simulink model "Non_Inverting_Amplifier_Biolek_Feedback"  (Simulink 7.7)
settings: Solver=ode113  StartTime=0.0  StopTime=10  RelTol=3e-14
libraries: fl_lib x7, nesl_utility x5, Memristor_lib x2

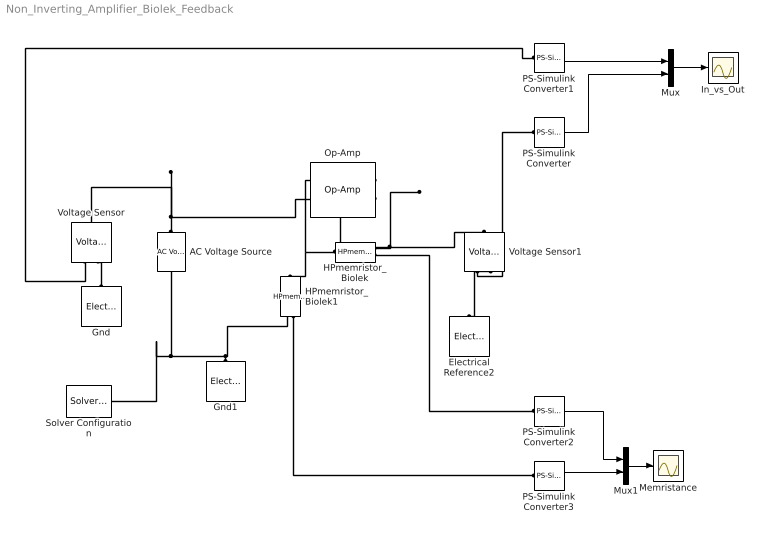
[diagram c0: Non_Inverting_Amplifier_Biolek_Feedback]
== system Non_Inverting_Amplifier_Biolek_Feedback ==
  AC Voltage Source : fl_lib/Electrical/Electrical Sources/AC Voltage Source  SystemSampleTime=-1  amp=1 V  shift=0 rad  omega=1 Hz  i_Log=off  v_Log=off  LocalVarNames=|i|v  LocalVarDescs=|i|v  LocalVarLogging=[0 0]
  Electrical Reference2 : fl_lib/Electrical/Electrical Elements/Electrical Reference  SystemSampleTime=-1  i_Log=off  LocalVarNames=|i  LocalVarDescs=|i  LocalVarLogging=0
  Gnd : fl_lib/Electrical/Electrical Elements/Electrical Reference  SystemSampleTime=-1  i_Log=off  LocalVarNames=|i  LocalVarDescs=|i  LocalVarLogging=0
  Gnd1 : fl_lib/Electrical/Electrical Elements/Electrical Reference  SystemSampleTime=-1  i_Log=off  LocalVarNames=|i  LocalVarDescs=|i  LocalVarLogging=0
  HPmemristor_Biolek : Memristor_lib/HPmemristor_Biolek  SystemSampleTime=-1  R_off=100 Ohm  R_on=2 Ohm  pp=10 m  u_v=1e-12 m^2/s/V  D=1e-8 m  w0=.01e-9 m  i_Log=off  v_Log=off  w_Log=off  F_Log=off  M_Log=off  LocalVarNames=|i|v|w|F|M  LocalVarDescs=|i|v|w|F|M  LocalVarLogging=[0 0 0 0 0]
  HPmemristor_Biolek1 : Memristor_lib/HPmemristor_Biolek  SystemSampleTime=-1  R_off=100 Ohm  R_on=2 Ohm  pp=10 m  u_v=1e-12 m^2/s/V  D=1e-8 m  w0=10e-9 m  i_Log=off  v_Log=off  w_Log=off  F_Log=off  M_Log=off  LocalVarNames=|i|v|w|F|M  LocalVarDescs=|i|v|w|F|M  LocalVarLogging=[0 0 0 0 0]
  In_vs_Out : Scope
  Memristance : Scope
  Mux : Mux  Inputs=2
  Mux1 : Mux  Inputs=2
  Op-Amp : fl_lib/Electrical/Electrical Elements/Op-Amp  SystemSampleTime=-1  i1_Log=off  v1_Log=off  outI_Log=off  LocalVarNames=|i1|v1|outI  LocalVarDescs=|i1|v1|outI  LocalVarLogging=[0 0 0]
  PS-Simulink Converter{,1..3} (4 alike) : nesl_utility/PS-Simulink Converter  SystemSampleTime=-1  PhysicalDomain=network_engine_domain  LeftPortType=input  RightPortType=output  SubClassName=ps_output  Unit=1  AffineConversion=off
  Solver Configuration : nesl_utility/Solver Configuration  SystemSampleTime=-1  PhysicalDomain=network_engine_domain  LeftPortType=input  RightPortType=generic  SubClassName=solver  Accelerate=off  Profile=off  ResidualTolerance=1e-9  MaxNonlinIter=3  MaxModeIter=2  DoFixedCost=off  UseLocalSampling=off  DoDC=off  LinearAlgebra=Sparse  LocalSolverSampleTime=.001  LocalSolverChoice=NE_BACKWARD_EULER_ADVANCER  UseLocalSolver=off
  Voltage Sensor : fl_lib/Electrical/Electrical Sensors/Voltage Sensor  SystemSampleTime=-1  i1_Log=off  v1_Log=off  LocalVarNames=|i1|v1  LocalVarDescs=|i1|v1  LocalVarLogging=[0 0]
  Voltage Sensor1 : fl_lib/Electrical/Electrical Sensors/Voltage Sensor  SystemSampleTime=-1  i1_Log=off  v1_Log=off  LocalVarNames=|i1|v1  LocalVarDescs=|i1|v1  LocalVarLogging=[0 0]
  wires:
  PS-Simulink Converter1/1 -> Mux/1
  PS-Simulink Converter/1 -> Mux/2
  Mux/1 -> In_vs_Out/1
  Mux1/1 -> Memristance/1
  PS-Simulink Converter2/1 -> Mux1/1
  PS-Simulink Converter3/1 -> Mux1/2
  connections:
  HPmemristor_Biolek/RConn1 -- Voltage Sensor1/LConn1 -- Op-Amp/RConn1
  HPmemristor_Biolek/LConn1 -- Op-Amp/LConn1 -- HPmemristor_Biolek1/LConn1
  Gnd1/LConn1 -- AC Voltage Source/RConn1 -- Solver Configuration/RConn1 -- HPmemristor_Biolek1/RConn1
  AC Voltage Source/LConn1 -- Voltage Sensor/LConn1 -- Op-Amp/LConn2
  Voltage Sensor1/RConn1 -- PS-Simulink Converter/LConn1
  Voltage Sensor/RConn1 -- PS-Simulink Converter1/LConn1
  Gnd/LConn1 -- Voltage Sensor/RConn2
  Electrical Reference2/LConn1 -- Voltage Sensor1/RConn2
  HPmemristor_Biolek1/RConn2 -- PS-Simulink Converter3/LConn1
  HPmemristor_Biolek/RConn2 -- PS-Simulink Converter2/LConn1
